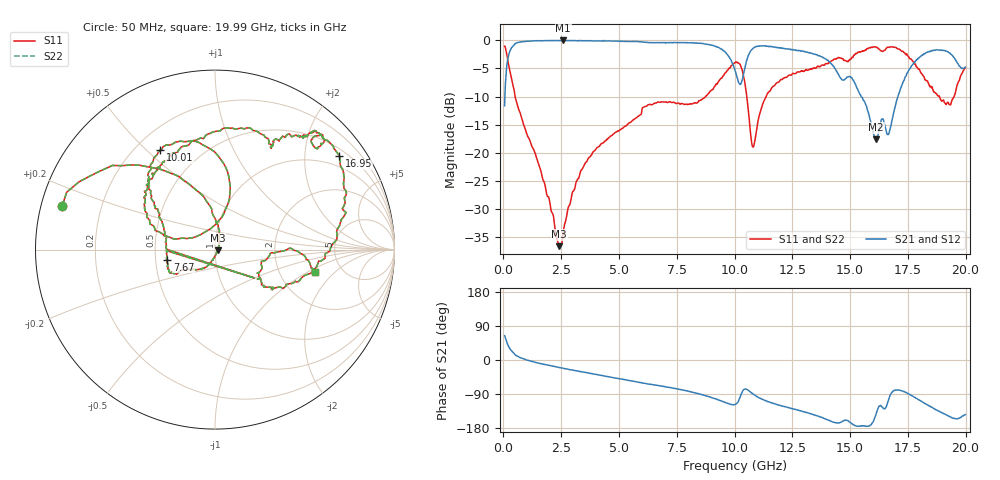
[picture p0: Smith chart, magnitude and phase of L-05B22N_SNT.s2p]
! Data Taken on a HP 8720C VNA using a shunt-through fixture with TRL* de-embedding
#	mhz	s	ma	r	50
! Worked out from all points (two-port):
!   998 points, 50 MHz to 19.99 GHz, reference 50 ohm
!   highest |S21| = -0.03 dB at 2.59 GHz (marker M1); lowest = -17.6 dB at 16.13 GHz (marker M2)
!   |S21| within 3 dB of the highest: 202.6 MHz to 9.781 GHz (9.578 GHz wide, 192 % of centre); 10.57 GHz to 13.82 GHz (3.252 GHz wide, 26.7 % of centre)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
!   lowest |S11| = -36.5 dB at 2.41 GHz (marker M3), VSWR 1.03, Z = 51.5 - j0.395 ohm
!   |S11| at or under -10 dB: 504.4 MHz to 8.742 GHz (8.238 GHz wide, 178 % of centre); 10.53 GHz to 11.36 GHz (833.2 MHz wide, 7.61 % of centre); 18.87 GHz to 19.5 GHz (630.6 MHz wide, 3.29 % of centre)
!   |S22| runs from -36.5 to -1.1 dB; largest |S21 - S12| = 0
!   S11 on the Smith chart (normalised r, x): 50 MHz: 0.06, +0.14; 7.67 GHz: 0.58, -0.07; 10.01 GHz: 0.30, +0.55; 16.95 GHz: 0.68, +2.85; 19.99 GHz: 3.20, -1.18
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50  0.8857 164.0  0.2622 64.1  0.2622 64.1  0.8857 164.0
230  0.5959 129.2  0.7444 34.9  0.7444 34.9  0.5959 129.2
570  0.281 100.5  0.9482 11.1  0.9482 11.1  0.281 100.5
2410  0.01488 -14.9  0.9945 -19.7  0.9945 -19.7  0.01488 -14.9
2590  0.02004 -65.3  0.9963 -21.9  0.9963 -21.9  0.02004 -65.3
3390  0.07105 -106.1  0.9912 -31.1  0.9912 -31.1  0.07105 -106.1
6710  0.2829 -152.6  0.9521 -67.3  0.9521 -67.3  0.2829 -152.6
7670  0.2724 -168.2  0.9511 -78.1  0.9511 -78.1  0.2724 -168.2
9110  0.3816 146.0  0.894 -101.3  0.894 -101.3  0.3816 146.0
10010  0.6328 119.0  0.5511 -117.8  0.5511 -117.8  0.6328 119.0
10030  0.6345 117.7  0.5326 -117.3  0.5326 -117.3  0.6345 117.7
10470  0.3905 78.1  0.5991 -76.5  0.5991 -76.5  0.3905 78.1
10810  0.1127 124.9  0.8519 -90.3  0.8519 -90.3  0.1127 124.9
11570  0.3648 159.1  0.8794 -112.6  0.8794 -112.6  0.3648 159.1
13350  0.5604 123.0  0.765 -142.9  0.765 -142.9  0.5604 123.0
15090  0.7049 60.0  0.4582 -168.9  0.4582 -168.9  0.7049 60.0
16130  0.8632 46.1  0.1322 -141.2  0.1322 -141.2  0.8632 46.1
16670  0.8682 46.2  0.1475 -104.1  0.1475 -104.1  0.8682 46.2
16950  0.8663 36.9  0.2556 -79.9  0.2556 -79.9  0.8663 36.9
18270  0.4434 -27.1  0.7727 -115.6  0.7727 -115.6  0.4434 -27.1
19310  0.2684 -15.3  0.7736 -149.3  0.7736 -149.3  0.2684 -15.3
19990  0.5721 -12.6  0.5769 -144.1  0.5769 -144.1  0.5721 -12.6
